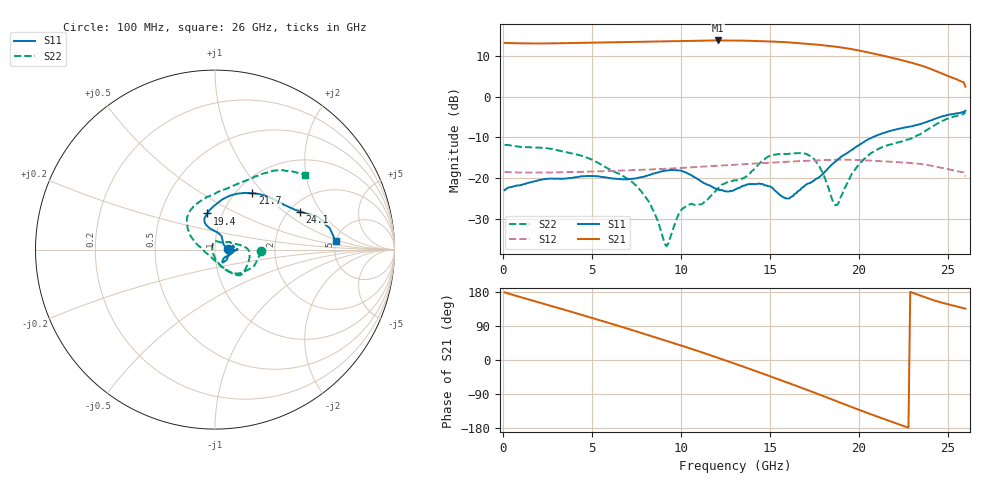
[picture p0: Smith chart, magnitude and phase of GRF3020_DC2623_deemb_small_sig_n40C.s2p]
!Keysight Technologies,N5245B,MY56052315,A.20.20.05
!Date: Tuesday, July 28, 2026 13:11:14
!Correction: S11(C  2-Port  )
!S21(C  2-Port  )
!S12(C  2-Port  )
!S22(C  2-Port  )
!S2P File: Measurements: S11, S21, S12, S22:
# Hz S  dB  R 50
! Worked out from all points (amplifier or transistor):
!   260 points, 100 MHz to 26 GHz, reference 50 ohm
!   highest |S21| = 13.9 dB at 12.1 GHz (marker M1)
!   |S21| within 3 dB of that: start of sweep to 20.6 GHz
!   unconditionally stable (mu >= 1): start of sweep to end of sweep
!   at 4.4 GHz: K = 1.16, MAG = 13.5 dB, |S12| = -18.5 dB
!   at 13.1 GHz: K = 1.04, MAG = 14.0 dB, |S12| = -16.7 dB
!   at 26 GHz: K = 1.46, MAG = 7.0 dB, |S12| = -19.6 dB
!   S11 on the Smith chart (normalised r, x): 100 MHz: 1.15, +0.00; 19.4 GHz: 0.85, +0.36; 21.7 GHz: 1.18, +0.87; 24.1 GHz: 2.26, +1.30; 26 GHz: 4.99, +0.83
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1e8  -22.96 1.3  13.26 178.5  -18.50 -0.8  -11.85 -2.0
2.3e9  -20.26 3.5  13.13 148.3  -18.63 -14.3  -12.55 -23.2
4.5e9  -19.53 6.5  13.27 118.2  -18.45 -27.8  -14.59 -45.5
6.7e9  -20.30 6.8  13.47 87.2  -18.13 -41.9  -19.33 -68.1
7.8e9  -19.73 -0.2  13.57 71.2  -17.94 -49.4  -23.35 -79.0
8.8e9  -18.50 -1.5  13.64 56.5  -17.75 -56.3  -31.72 -114.0
9.2e9  -18.12 -0.5  13.68 50.6  -17.68 -59.1  -36.73 -169.9
1e10  -18.15 1.8  13.74 38.6  -17.50 -64.8  -27.96 104.4
1.07e10  -19.58 -5.7  13.80 27.9  -17.31 -69.9  -26.50 79.9
1.21e10  -22.83 -31.7  13.86 5.6  -16.94 -80.9  -22.51 33.2
1.31e10  -22.70 -54.0  13.84 -10.6  -16.68 -89.0  -20.56 24.9
1.42e10  -21.51 -49.8  13.74 -29.1  -16.40 -98.5  -17.44 12.1
1.55e10  -23.83 1.3  13.53 -51.1  -16.06 -110.1  -14.09 -12.5
1.65e10  -23.67 50.2  13.27 -68.3  -15.85 -119.6  -13.87 -37.1
1.74e10  -20.81 75.5  12.93 -84.1  -15.68 -128.4  -14.94 -51.7
1.87e10  -15.88 111.0  12.34 -107.6  -15.48 -142.6  -26.68 -128.7
1.94e10  -13.72 101.9  11.88 -120.4  -15.47 -150.3  -20.80 168.0
2.05e10  -10.54 78.0  10.96 -139.9  -15.65 -162.5  -14.49 143.4
2.17e10  -8.48 56.4  9.78 -160.4  -15.93 -175.4  -11.83 123.1
2.29e10  -7.32 40.3  8.47 179.6  -16.27 171.6  -10.33 93.1
2.41e10  -5.74 24.1  6.78 159.5  -16.96 157.5  -7.47 65.5
2.6e10  -3.43 3.9  2.50 135.4  -19.60 141.9  -3.73 39.9
